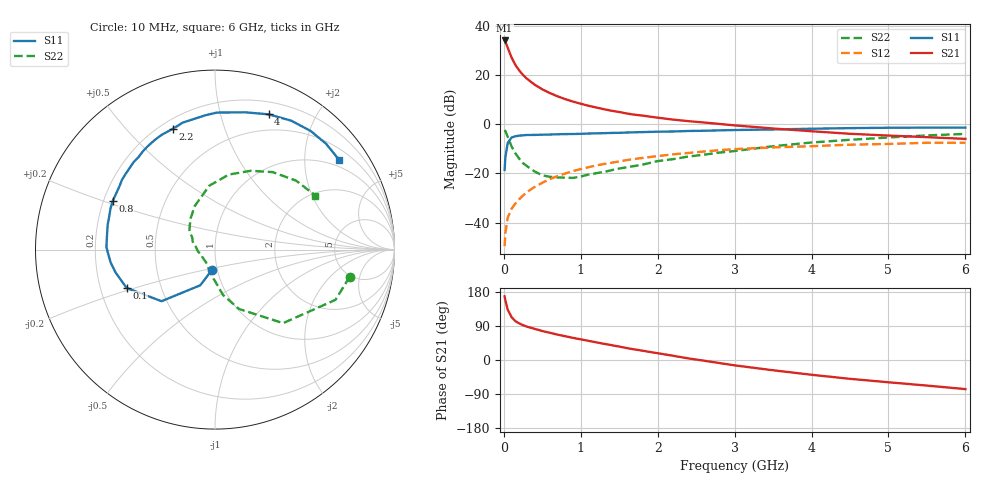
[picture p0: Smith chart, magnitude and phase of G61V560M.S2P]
! SIEMENS Small Signal Semiconductors
! BFG193
! Si NPN RF Bipolar Junction Transistor in SOT223
! VCE = 1.5 V  IC = 60 mA
! Common Emitter S-Parameters:  August  1996
# GHz  S  MA  R  50
!  f  S11  S21  S12  S22
! GHz  MAG  ANG  MAG  ANG  MAG  ANG  MAG  ANG
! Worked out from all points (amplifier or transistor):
!   36 points, 10 MHz to 6 GHz, reference 50 ohm
!   highest |S21| = 34.1 dB at 10 MHz (marker M1)
!   |S21| within 3 dB of that: start of sweep to 50.71 MHz
!   unconditionally stable (mu >= 1): start of sweep to 13.28 MHz; 223.8 MHz to 2.942 GHz; 3.144 GHz to 3.875 GHz
!   at 250 MHz: K = 1.02, MAG = 23.6 dB, |S12| = -29.0 dB
!   at 1.4 GHz: K = 1.11, MAG = 8.6 dB, |S12| = -15.7 dB
!   at 6 GHz: K = 1.00, MSG = 0.8 dB, |S12| = -7.5 dB
!   S11 on the Smith chart (normalised r, x): 10 MHz: 0.94, -0.22; 100 MHz: 0.31, -0.19; 800 MHz: 0.24, +0.21; 2.2 GHz: 0.25, +0.68; 4 GHz: 0.32, +1.42; 6 GHz: 0.78, +2.89
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0.01  0.1175 -99.3  50.8 168.0  0.0033 80.8  0.7658 -11.3
0.02  0.2149 -112.4  47.86 157.3  0.0062 74.8  0.7275 -22.6
0.05  0.4138 -136.0  36.2 132.9  0.0125 63.8  0.5585 -47.2
0.1  0.5367 -156.5  22.95 113.4  0.019 62.1  0.356 -68.1
0.15  0.569 -167.2  16.13 102.5  0.0244 62.5  0.2557 -80.1
0.2  0.5859 -173.0  12.46 96.6  0.0298 64.7  0.1996 -85.9
0.25  0.5958 -177.8  10.06 91.8  0.0355 66.2  0.1609 -93.2
0.3  0.6051 178.6  8.464 88.1  0.0417 67.3  0.1409 -98.5
0.4  0.6069 172.6  6.401 82.2  0.053 67.4  0.1091 -109.2
0.5  0.6136 167.0  5.141 76.5  0.0644 66.5  0.0914 -119.1
0.6  0.6175 162.7  4.305 71.7  0.0769 65.2  0.0852 -128.1
0.7  0.6261 158.3  3.701 66.9  0.0883 64.2  0.0828 -138.6
0.8  0.631 154.4  3.238 62.6  0.0996 62.0  0.0816 -149.6
1.1  0.6479 143.2  2.378 50.6  0.1336 56.2  0.0945 -173.0
1.6  0.6789 126.3  1.652 31.4  0.1867 44.5  0.1336 159.0
2.2  0.7129 109.2  1.243 11.2  0.2439 30.0  0.1947 136.2
2.8  0.7513 93.7  1.016 -8.0  0.2967 15.3  0.265 116.0
3.5  0.7831 77.6  0.82 -27.1  0.338 -2.7  0.3574 95.1
4  0.8107 68.4  0.721 -39.0  0.3577 -12.6  0.4254 79.5
4.5  0.8345 59.4  0.64 -49.7  0.3842 -22.7  0.4826 65.5
5.5  0.8548 43.6  0.546 -67.5  0.4198 -45.6  0.5929 40.4
6  0.8532 36.0  0.504 -76.8  0.4196 -58.7  0.6355 28.3
